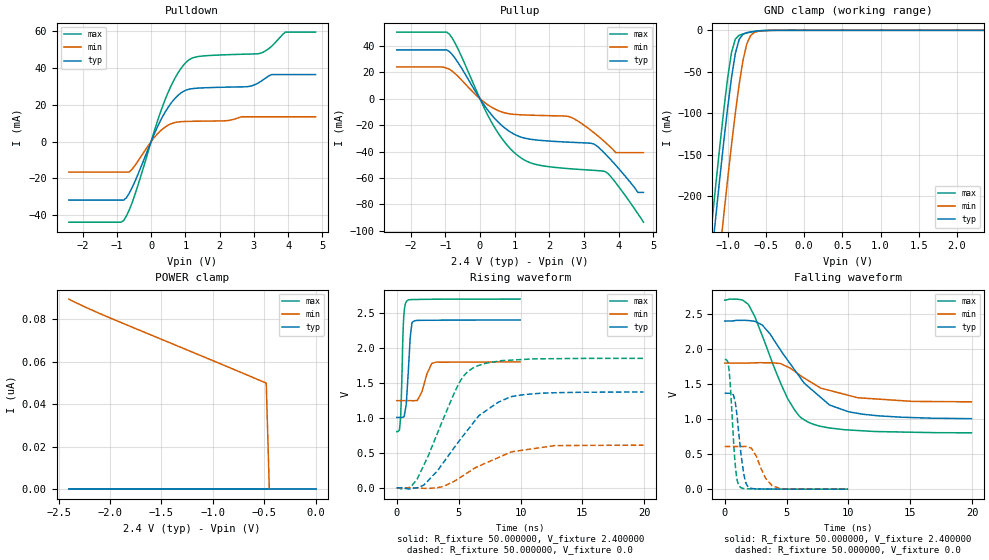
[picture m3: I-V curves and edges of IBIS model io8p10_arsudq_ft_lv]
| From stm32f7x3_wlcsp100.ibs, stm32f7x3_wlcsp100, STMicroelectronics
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|   Model io8p10_arsudq_ft_lv
[Model]  io8p10_arsudq_ft_lv
Model_type I/O
Polarity   Non-Inverting
Enable   Active-Low
Vinl =   0.720000V
Vinh =   1.680000V
Vmeas =  1.200000V
Cref =   40.000000pF
Rref =   100.000000M
Vref =   0.0V
C_comp   2.239000pF   2.178700pF   2.334000pF
[Temperature Range]   25.000000   0.125000k   -40.000000
[Pullup Reference]   2.400000V   1.800000V   2.700000V
[Pulldown Reference]   0.0V   0.0V   0.0V
[POWER Clamp Reference]   2.400000V   1.800000V   2.700000V
[GND Clamp Reference]   0.0V   0.0V   0.0V
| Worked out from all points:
|   slope of the pulldown table from 0 to 0.36 V, typ, clamps not added: 25 ohm
|   slope of the pullup table from 0 to 0.36 V, typ, clamps not added: 27.7 ohm
|   GND clamp passes 1 mA (typ) near -0.62 V on its own axis
|   rising waveform, R_fixture 50.000000, V_fixture 2.400000: 20-80 % time 277ps typ, 616ps min, 182ps max; typ from 1.01 V to 2.4 V
|   rising waveform, R_fixture 50.000000, V_fixture 0.0: 20-80 % time 3.74ns typ, 4.02ns min, 2.67ns max; typ from 0 V to 1.37 V
|   falling waveform, R_fixture 50.000000, V_fixture 2.400000: 20-80 % time 3.91ns typ, 4.01ns min, 2.72ns max; typ from 2.4 V to 1.01 V
|   falling waveform, R_fixture 50.000000, V_fixture 0.0: 20-80 % time 529ps typ, 978ps min, 383ps max; typ from 1.37 V to 0 V
[Pulldown]
|Voltage   I(typ)   I(min)   I(max)
-2.4V     -31.73mA   -16.51mA   -43.74mA
-800mV    -31.73mA   -16.51mA   -42.87mA
-480mV    -21.98mA   -13.17mA   -29.21mA
80mV      3.63mA     1.966mA    5.014mA
480mV     18.16mA    8.738mA    26.02mA
800mV     25.38mA    10.72mA    37.77mA
1.12V     28.53mA    11.02mA    44.6mA
2.8V      29.84mA    13.49mA    47.53mA
3.2V      32.65mA    13.49mA    48.05mA
3.52V     36.43mA    13.49mA    51.84mA
3.92V     36.43mA    13.49mA    59.49mA
4.8V      36.43mA    13.49mA    59.49mA
[Pullup]
|Voltage   I(typ)   I(min)   I(max)
-2.4V     36.91mA    24.04mA    50.37mA
-960mV    36.91mA    23.05mA    50.37mA
-640mV    27.65mA    17.03mA    38mA
320mV     -11.75mA   -6.207mA   -17.08mA
960mV     -26.47mA   -11.82mA   -40.02mA
1.52V     -30.88mA   -12.51mA   -49.05mA
2.56V     -32.88mA   -13.48mA   -52.9mA
3.28V     -34.19mA   -25.52mA   -54.18mA
3.6V      -41.31mA   -32.62mA   -54.97mA
3.92V     -50.32mA   -40.8mA    -63.62mA
4.56V     -70.9mA    -40.8mA    -87.08mA
4.72V     -70.9mA    -40.8mA    -93.4mA
[GND_clamp]
|Voltage   I(typ)   I(min)   I(max)
-2.4V     -1.424A    -1.508A    -1.393A
-1.25V    -311.2mA   -401.9mA   -273.3mA
-1.2V     -265.4mA   -356.1mA   -227.2mA
-1.15V    -220.4mA   -310.8mA   -181.9mA
-1.1V     -176.3mA   -266.2mA   -137.9mA
-1.05V    -133.8mA   -222.5mA   -95.87mA
-950mV    -57.3mA    -138.9mA   -26.98mA
-900mV    -28.27mA   -100.4mA   -10.59mA
-850mV    -11.01mA   -65.54mA   -5.958mA
-750mV    -2.834mA   -16.5mA    -3.178mA
-600mV    -750uA     -1.164mA   -738.3uA
2.35V     0A         0A         0A
[POWER_clamp]
|Voltage   I(typ)   I(min)   I(max)
-2.4V     0A         89.62nA    0A
-2.04V    0A         81.57nA    0A
-480mV    0A         50.01nA    0A
-450mV    0A         0A         0A
0V        0A         0A         0A
[Ramp]
| variable   typ   min   max
dV/dt_r  0.82206/3.73978n   0.36598/4.02494n   1.11102/2.66595n
dV/dt_f  0.83268/3.90784n   0.33198/4.05694n   1.13662/2.72279n
R_load = 50.000000
[Rising Waveform]
R_fixture= 50.000000
V_fixture= 2.400000
V_fixture_min= 1.800000
V_fixture_max= 2.700000
|time   V(typ)   V(min)   V(max)
0s        1.006V     1.247V     804.6mV
220.2ps   1.006V     1.247V     831.3mV
300.3ps   1.006V     1.247V     989.8mV
560.6ps   1.015V     1.247V     2.439V
820.8ps   1.347V     1.247V     2.675V
1.081ns   2.139V     1.247V     2.691V
1.341ns   2.381V     1.245V     2.693V
2.042ns   2.395V     1.38V      2.695V
2.843ns   2.397V     1.779V     2.697V
9.97ns    2.4V       1.8V       2.699V
[Rising Waveform]
R_fixture= 50.000000
V_fixture= 0.0
V_fixture_min= 0.0
V_fixture_max= 0.0
|time   V(typ)   V(min)   V(max)
0s        168.7uV    66.34uV    586uV
1.121ns   -14.77mV   125.1uV    12.42mV
1.642ns   534.1uV    -516.3uV   122.2mV
3.283ns   242.7mV    2.469mV    780.4mV
5.005ns   662.9mV    134.6mV    1.491V
6.206ns   934.6mV    271.3mV    1.718V
8.168ns   1.221V     429.7mV    1.81V
9.57ns    1.314V     522.5mV    1.83V
12.77ns   1.359V     604.1mV    1.847V
19.94ns   1.37V      609mV      1.851V
[Falling Waveform]
R_fixture= 50.000000
V_fixture= 2.400000
V_fixture_min= 1.800000
V_fixture_max= 2.700000
|time   V(typ)   V(min)   V(max)
0s        2.4V       1.8V       2.699V
1.441ns   2.41V      1.8V       2.7V
1.922ns   2.407V     1.801V     2.635V
3.043ns   2.342V     1.805V     2.187V
5.085ns   1.841V     1.745V     1.294V
6.046ns   1.607V     1.632V     1.04V
6.767ns   1.461V     1.55V      955.1mV
8.488ns   1.2V       1.409V     873.4mV
10.05ns   1.103V     1.337V     844.5mV
19.94ns   1.006V     1.247V     804.6mV
[Falling Waveform]
R_fixture= 50.000000
V_fixture= 0.0
V_fixture_min= 0.0
V_fixture_max= 0.0
|time   V(typ)   V(min)   V(max)
0s        1.37V      609mV      1.851V
340.3ps   1.37V      609mV      1.721V
440.4ps   1.37V      609mV      1.523V
700.7ps   1.346V     608.9mV    729.8mV
940.9ps   1.127V     608.7mV    199.9mV
1.241ns   625mV      608.5mV    32.65mV
1.682ns   105.8mV    610.3mV    6.466mV
2.042ns   17.92mV    591.4mV    3.997mV
3.844ns   1.622mV    48.6mV     1.662mV
9.97ns    168.7uV    66.34uV    586uV
